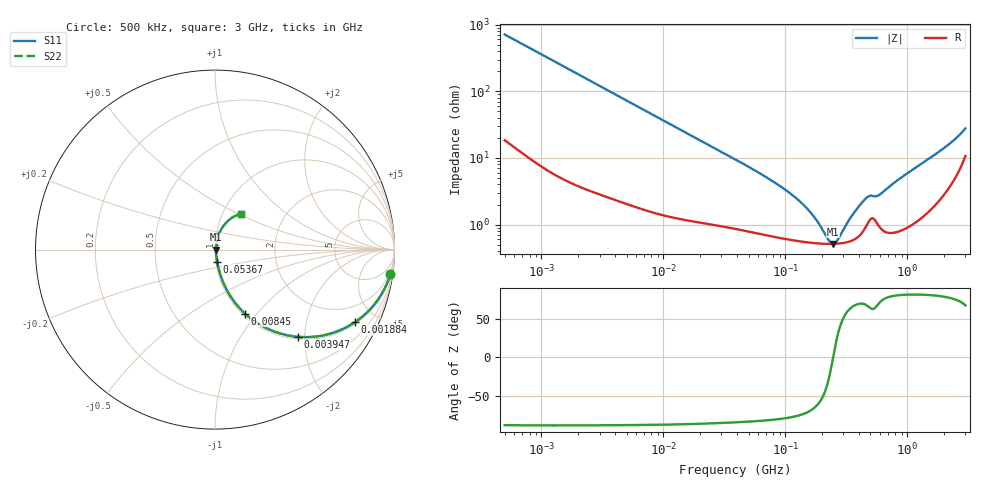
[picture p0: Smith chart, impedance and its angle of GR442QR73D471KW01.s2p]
!Murata Part Number: GR442QR73D471KW01
!These Parameters are Measured in Series Mode Connection
!Data Generated on Mar 13, 2026
!  o--ll--o
!Port1  Port2
!  o------o
!Operation Temp=25[degC], DC Bias Voltage=0[V]
!Freq. Start=500[kHz] Stop=3[GHz] 401[Steps]
# Hz S RI R 50
!Freq.(Hz) S11(Real) S11(Imag) S21(Real) S21(Imag) S12(Real) S12(Imag) S22(Real) S22(Imag)
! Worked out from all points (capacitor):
!   401 points, 500 kHz to 3 GHz, reference 50 ohm
!   read as one part in series: C = 445 pF near 522.2 kHz
!   lowest |Z| = 514 mohm at 246 MHz (marker M1)
!   series resonance near 247.2 MHz, so ESL is about 930 pH
!   S11 on the Smith chart (normalised r, x): 500 kHz: 1, -14; 1.884 MHz: 1.08, -3.84; 3.947 MHz: 1.05, -1.84; 8.45 MHz: 1.03, -0.87; 53.67 MHz: 1.02, -0.14; 3 GHz: 1.21, +0.51
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500000  0.9773 -0.1365  0.0227 0.1365  0.0227 0.1365  0.9773 -0.1365
1070430  0.9141 -0.2702  0.0859 0.2702  0.0859 0.2702  0.9141 -0.2702
1884248  0.7815 -0.403  0.2185 0.403  0.2185 0.403  0.7815 -0.403
2146893  0.7352 -0.4307  0.2648 0.4307  0.2648 0.4307  0.7352 -0.4307
3947125  0.4608 -0.4858  0.5392 0.4858  0.5392 0.4858  0.4608 -0.4858
8450242  0.1673 -0.3564  0.8327 0.3564  0.8327 0.3564  0.1673 -0.3564
9218297  0.1459 -0.3355  0.8541 0.3355  0.8541 0.3355  0.1459 -0.3355
1.658349e7  0.0569 -0.2075  0.9431 0.2075  0.9431 0.2075  0.0569 -0.2075
3.958139e7  0.0169 -0.0909  0.9831 0.0909  0.9831 0.0909  0.0169 -0.0909
5.366935e7  0.0121 -0.0667  0.9879 0.0667  0.9879 0.0667  0.0121 -0.0667
1.076412e8  0.00677 -0.0293  0.9932 0.0293  0.9932 0.0293  0.00677 -0.0293
1.662976e8  0.00545 -0.0131  0.9946 0.0131  0.9946 0.0131  0.00545 -0.0131
2.254869e8  0.00511 -0.003  0.9949 0.003  0.9949 0.003  0.00511 -0.003
2.459817e8  0.00511 -0.000161  0.9949 0.000161  0.9949 0.000161  0.00511 -0.000161
2.683393e8  0.00516 0.00271  0.9948 -0.00271  0.9948 -0.00271  0.00516 0.00271
3.483604e8  0.0058 0.0118  0.9942 -0.0118  0.9942 -0.0118  0.0058 0.0118
4.42515e8  0.00868 0.0213  0.9913 -0.0213  0.9913 -0.0213  0.00868 0.0213
4.933497e8  0.0121 0.0238  0.9879 -0.0238  0.9879 -0.0238  0.0121 0.0238
5.871079e8  0.01 0.0255  0.99 -0.0255  0.99 -0.0255  0.01 0.0255
7.140462e8  0.00872 0.0358  0.9913 -0.0358  0.9913 -0.0358  0.00872 0.0358
1.900064e9  0.0393 0.1206  0.9607 -0.1206  0.9607 -0.1206  0.0393 0.1206
3e9  0.1427 0.1984  0.8573 -0.1984  0.8573 -0.1984  0.1427 0.1984
